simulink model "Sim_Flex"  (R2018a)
settings: Solver=ode113  StartTime=0.0  StopTime=20  FixedStep=0.0001  RelTol=1e-5  EnableMultiTasking=on
InitFcn:
  | init
StopFcn:
  | pl
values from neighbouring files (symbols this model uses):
  d2r = pi/180    (= 0.0174532925199)    [init.m]    (also in LQR_Design.m)
  Kr = Kq; Kr(3:4)=-Kq(3:4)    [init.m]
  Wf = 20    [init.m]
undefined symbols (not defined in the file or in its folder): Av, Bv, Cv, Dv, Kq, TVC
libraries: Actuator_Lib x16

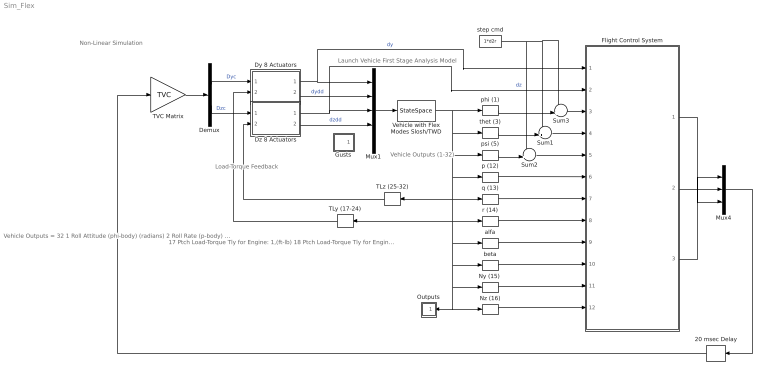
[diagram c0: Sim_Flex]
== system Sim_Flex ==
  note: Load-Torque Feedback
  note: 17 Ptch Load-Torque Tly for Engine: 1,(ft-lb) 18 Ptch Load-Torque Tly for Engine: 2,(ft-lb) 19 Ptch Load-Torque Tly for Engine: 3,(ft-lb) 20 Ptch Load-Torque Tly for Engine: 4,(ft-lb) 21 Ptch Load-Torque Tly for Engine: 5,(ft-lb) 22 Ptch Load-Torque Tly for Engine: 6,(ft-lb) 23 Ptch Load-Torque Tly for Engine: 7,(ft-lb) 24 Ptch Load-Torque Tly for Engine: 8,(ft-lb) 25 Yaw Load-Torque Tlz for Engine: 1,(ft-lb) 26 Yaw Load-Torque Tlz for Engine: 2,(ft-lb) 27 Yaw Load-Torque Tlz for Engine: 3,(ft-lb) 28 Yaw Load-Torque Tlz for Engine: 4,(ft-lb) 29 Yaw Load-Torque Tlz for Engine: 5,(ft-lb) 30 Yaw Load-Torque Tlz for Engine: 6,(ft-lb) 31 Yaw Load-Torque Tlz for Engine: 7,(ft-lb) 32 Yaw Load-Torque Tlz for Engine: 8,(ft-lb)
  note: Vehicle Outputs = 32 1 Roll Attitude (phi-body) (radians) 2 Roll Rate (p-body) (rad/sec) 3 Pitch Attitude (thet-bdy) (radians) 4 Pitch Rate (q-body) (rad/sec) 5 Yaw Attitude (psi-body) (radians) 6 Yaw Rate (r-body) (rad/sec) 7 Angle of attack, alfa, (radians) 8 Angle of sideslip, beta, (radian) 9 Change in Altitude, delta-h, (feet) 10 Forward Acceleration (V-dot) (ft/sec) 11 Cross Range Velocity (Vcr) (ft/sec) 12 Rate-Gyro # 1, Roll Rate (Body) (rad/sec) 13 Rate-Gyro # 2, Pitch Rate (Body) (rad/sec) 14 Rate-Gyro # 3, Yaw Rate (Body) (rad/sec) 15 Accelerom # 1, (along Y), (ft/sec^2) Translat. Accelerat. 16 Accelerom # 2, (along Z), (ft/sec^2) Translat. Accelerat.
  note: Vehicle Outputs (1-32)
  note: Non-Linear Simulation
  note: Launch Vehicle First Stage Analysis Model
  20 msec Delay : TransportDelay  DelayTime="[1  1  1]*0.02"  InitialOutput="[0  0  0]"  PadeOrder=2
  Demux : Demux  Outputs=[8, 8]
  Dy 8 Actuators : Subsystem
  Dz 8 Actuators : Subsystem
  Flight Control System : Subsystem
  Gusts : Subsystem
  Mux1 : Mux  Inputs=[8, 8, 8, 8, 1]
  Mux4 : Mux  Inputs=3
  "Ny (15) " : Selector  InputPortWidth=32  IndexOptions=Index vector (dialog)  Indices=[15]  OutputSizes=1
  Nz (16) : Selector  InputPortWidth=32  IndexOptions=Index vector (dialog)  Indices=[16]  OutputSizes=1
  Outputs : Subsystem
  Sum1 : Sum  Inputs=-+|
  Sum2 : Sum  Inputs=-+|
  Sum3 : Sum  Inputs=-+|
  TLy (17-24) : Selector  InputPortWidth=32  IndexOptions=Index vector (dialog)  Indices=[17:24]  OutputSizes=1
  TLz (25-32) : Selector  InputPortWidth=32  IndexOptions=Index vector (dialog)  Indices=[25:32]  OutputSizes=1
  TVC Matrix : Gain  Gain=TVC  Multiplication=Matrix(K*u)
  Vehicle with Flex Modes Slosh/TWD : StateSpace  A=Av  B=Bv  C=Cv  D=Dv  InitialCondition=0
  alfa : Selector  InputPortWidth=32  IndexOptions=Index vector (dialog)  Indices=[7]  OutputSizes=1
  beta : Selector  InputPortWidth=32  IndexOptions=Index vector (dialog)  Indices=[8]  OutputSizes=1
  p (12) : Selector  InputPortWidth=32  IndexOptions=Index vector (dialog)  Indices=[12]  OutputSizes=1
  phi (1) : Selector  InputPortWidth=32  IndexOptions=Index vector (dialog)  Indices=[1]  OutputSizes=1
  psi (5) : Selector  InputPortWidth=32  IndexOptions=Index vector (dialog)  Indices=[5]  OutputSizes=1
  q (13) : Selector  InputPortWidth=32  IndexOptions=Index vector (dialog)  Indices=[13]  OutputSizes=1
  r (14) : Selector  InputPortWidth=32  IndexOptions=Index vector (dialog)  Indices=[14]  OutputSizes=1
  step cmd : Constant  Value=1*d2r
  thet (3) : Selector  InputPortWidth=32  IndexOptions=Index vector (dialog)  Indices=[3]  OutputSizes=1
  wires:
  Mux1/1 -> Vehicle with Flex Modes Slosh/TWD/1
  Dy 8 Actuators/2(dydd) -> Mux1/2  "dydd"
  Dz 8 Actuators/2(dzdd) -> Mux1/4  "dzdd"
  Demux/1 -> Dy 8 Actuators/1(dy-com)  "Dyc"
  Dy 8 Actuators/1(DY) -> Flight Control System/1(dy), Mux1/1  "dy"
  Dz 8 Actuators/1(DZ) -> Flight Control System/2(dz), Mux1/3  "dz"
  Demux/2 -> Dz 8 Actuators/1(dz-com)  "Dzc"
  TLy (17-24)/1 -> Dy 8 Actuators/2(TLY)
  TLz (25-32)/1 -> Dz 8 Actuators/2(TLZ)
  Vehicle with Flex Modes Slosh/TWD/1 -> TLz (25-32)/1, "Ny (15) "/1, Outputs/1(in), Nz (16)/1, beta/1, alfa/1, TLy (17-24)/1, r (14)/1, q (13)/1, p (12)/1, psi (5)/1, thet (3)/1, phi (1)/1
  r (14)/1 -> Flight Control System/8(r)
  q (13)/1 -> Flight Control System/7(q)
  p (12)/1 -> Flight Control System/6(p)
  TVC Matrix/1 -> Demux/1
  alfa/1 -> Flight Control System/9(alfa)
  beta/1 -> Flight Control System/10(beta)
  "Ny (15) "/1 -> Flight Control System/11(NY)
  Nz (16)/1 -> Flight Control System/12(NZ)
  Flight Control System/2(DQ_tvc) -> Mux4/2
  Flight Control System/1(DP_tvc) -> Mux4/1
  Flight Control System/3(DR_tvc) -> Mux4/3
  Mux4/1 -> 20 msec Delay/1
  Sum3/1 -> Flight Control System/3(phi)
  phi (1)/1 -> Sum3/2
  Sum1/1 -> Flight Control System/4(thet)
  thet (3)/1 -> Sum1/2
  psi (5)/1 -> Sum2/2
  Sum2/1 -> Flight Control System/5(psi)
  step cmd/1 -> Sum3/1, Sum1/1, Sum2/1
  20 msec Delay/1 -> TVC Matrix/1

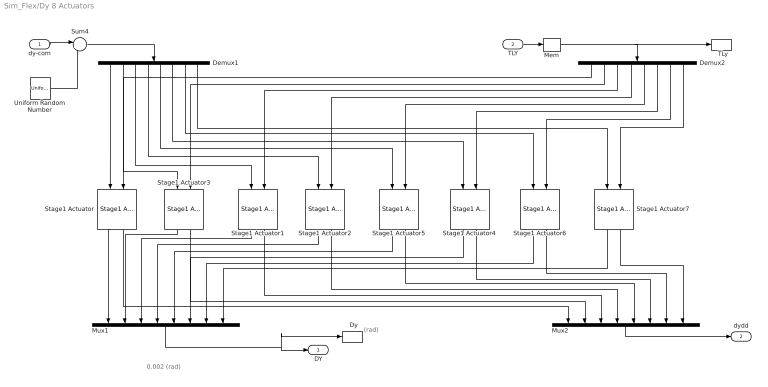
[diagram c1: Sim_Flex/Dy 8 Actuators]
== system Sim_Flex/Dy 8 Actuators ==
  note: (rad)
  note: 0.002 (rad)
  dy-com : Inport
  TLY : Inport  Port=2
  "  Dy" : ToWorkspace  VariableName=DY  SampleTime=-1
  "  TLy" : ToWorkspace  VariableName=TLy  SampleTime=-1
  Demux1 : Demux  Outputs=8
  Demux2 : Demux  Outputs=8
  Mem : Memory
  Mux1 : Mux  Inputs=8
  Mux2 : Mux  Inputs=8
  Stage1 Actuator{,1..7} (8 alike) : Actuator_Lib/Stage1 Actuator
  Sum4 : Sum  Inputs=|++
  Uniform Random Number : UniformRandomNumber  Minimum=[-1 -1 -1 -1 -1 -1 -1 -1]*0.002  Maximum=[1 1 1 1 1 1 1 1]*0.002  Seed=[10,11,12,13, 15,16,17,18]  SampleTime=0.001
  DY : Outport
  dydd : Outport  Port=2
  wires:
  Mux1/1 -> "  Dy"/1, DY/1
  TLY/1 -> Mem/1
  Mux2/1 -> dydd/1
  Stage1 Actuator2/1 -> Mux1/4
  Demux1/5 -> Stage1 Actuator5/1
  Stage1 Actuator4/2 -> Mux2/6
  Stage1 Actuator/1 -> Mux1/1
  Demux1/4 -> Stage1 Actuator2/1
  Stage1 Actuator7/1 -> Mux1/8
  Stage1 Actuator5/2 -> Mux2/5
  Stage1 Actuator5/1 -> Mux1/5
  Demux2/4 -> Stage1 Actuator2/2
  Demux2/6 -> Stage1 Actuator4/2
  Demux2/7 -> Stage1 Actuator6/2
  Stage1 Actuator1/2 -> Mux2/3
  Demux2/2 -> Stage1 Actuator3/2
  Stage1 Actuator2/2 -> Mux2/4
  Demux1/3 -> Stage1 Actuator1/1
  Stage1 Actuator6/2 -> Mux2/7
  Stage1 Actuator/2 -> Mux2/1
  Stage1 Actuator7/2 -> Mux2/8
  Stage1 Actuator3/2 -> Mux2/2
  Demux1/2 -> Stage1 Actuator3/1
  Demux1/7 -> Stage1 Actuator6/1
  Demux1/8 -> Stage1 Actuator7/1
  Stage1 Actuator3/1 -> Mux1/2
  Demux2/5 -> Stage1 Actuator5/2
  Demux1/1 -> Stage1 Actuator/1
  Demux2/1 -> Stage1 Actuator/2
  Stage1 Actuator6/1 -> Mux1/7
  Demux2/8 -> Stage1 Actuator7/2
  Demux2/3 -> Stage1 Actuator1/2
  Stage1 Actuator4/1 -> Mux1/6
  Stage1 Actuator1/1 -> Mux1/3
  Demux1/6 -> Stage1 Actuator4/1
  Mem/1 -> Demux2/1, "  TLy"/1
  dy-com/1 -> Sum4/1
  Uniform Random Number/1 -> Sum4/2
  Sum4/1 -> Demux1/1

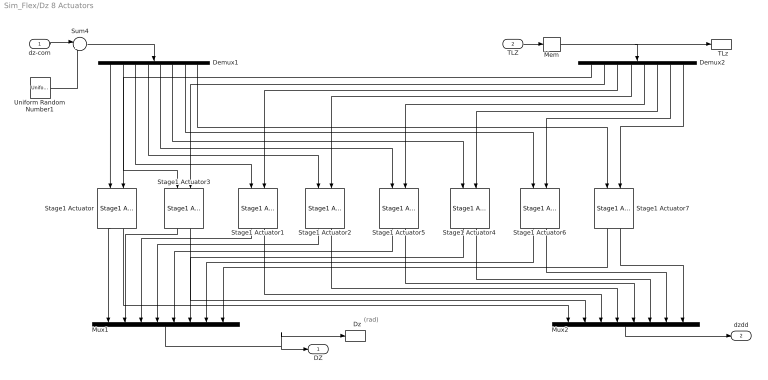
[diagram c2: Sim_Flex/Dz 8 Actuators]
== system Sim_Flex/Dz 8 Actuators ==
  note: (rad)
  dz-com : Inport
  TLZ : Inport  Port=2
  "  Dz" : ToWorkspace  VariableName=DZ  SampleTime=-1
  "  TLz" : ToWorkspace  VariableName=TLz  SampleTime=-1
  Demux1 : Demux  Outputs=8
  Demux2 : Demux  Outputs=8
  Mem : Memory
  Mux1 : Mux  Inputs=8
  Mux2 : Mux  Inputs=8
  Stage1 Actuator{,1..7} (8 alike) : Actuator_Lib/Stage1 Actuator
  Sum4 : Sum  Inputs=|++
  Uniform Random Number1 : UniformRandomNumber  Minimum=[-1 -1 -1 -1 -1 -1 -1 -1]*0.002  Maximum=[1 1 1 1 1 1 1 1]*0.002  Seed=[10,11,12,13, 15,16,17,18]  SampleTime=0.001
  DZ : Outport
  dzdd : Outport  Port=2
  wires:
  Mux1/1 -> "  Dz"/1, DZ/1
  TLZ/1 -> Mem/1
  Mux2/1 -> dzdd/1
  Stage1 Actuator2/1 -> Mux1/4
  Demux1/5 -> Stage1 Actuator5/1
  Stage1 Actuator4/2 -> Mux2/6
  Stage1 Actuator/1 -> Mux1/1
  Demux1/4 -> Stage1 Actuator2/1
  Stage1 Actuator7/1 -> Mux1/8
  Stage1 Actuator5/2 -> Mux2/5
  Stage1 Actuator5/1 -> Mux1/5
  Demux2/4 -> Stage1 Actuator2/2
  Demux2/6 -> Stage1 Actuator4/2
  Demux2/7 -> Stage1 Actuator6/2
  Stage1 Actuator1/2 -> Mux2/3
  Demux2/2 -> Stage1 Actuator3/2
  Stage1 Actuator2/2 -> Mux2/4
  Demux1/3 -> Stage1 Actuator1/1
  Stage1 Actuator6/2 -> Mux2/7
  Stage1 Actuator/2 -> Mux2/1
  Stage1 Actuator7/2 -> Mux2/8
  Stage1 Actuator3/2 -> Mux2/2
  Demux1/2 -> Stage1 Actuator3/1
  Demux1/7 -> Stage1 Actuator6/1
  Demux1/8 -> Stage1 Actuator7/1
  Stage1 Actuator3/1 -> Mux1/2
  Demux2/5 -> Stage1 Actuator5/2
  Demux1/1 -> Stage1 Actuator/1
  Demux2/1 -> Stage1 Actuator/2
  Stage1 Actuator6/1 -> Mux1/7
  Demux2/8 -> Stage1 Actuator7/2
  Demux2/3 -> Stage1 Actuator1/2
  Stage1 Actuator4/1 -> Mux1/6
  Stage1 Actuator1/1 -> Mux1/3
  Demux1/6 -> Stage1 Actuator4/1
  Mem/1 -> Demux2/1, "  TLz"/1
  dz-com/1 -> Sum4/1
  Uniform Random Number1/1 -> Sum4/2
  Sum4/1 -> Demux1/1

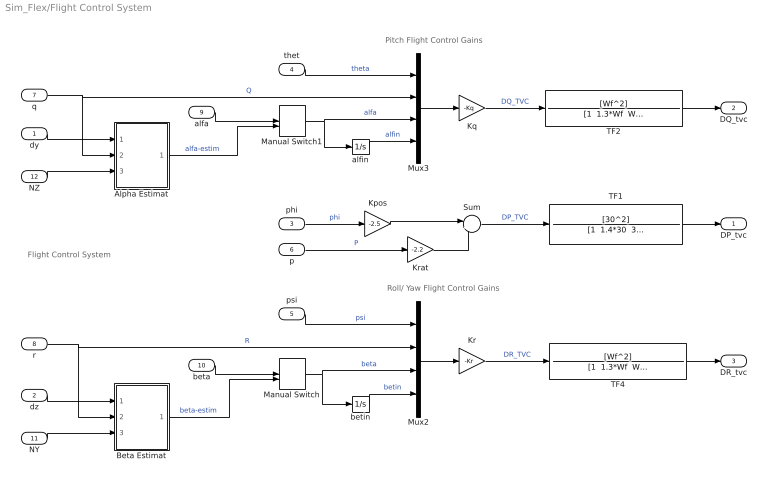
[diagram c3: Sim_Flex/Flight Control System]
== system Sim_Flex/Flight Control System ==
  note: Pitch Flight Control Gains
  note: Roll/ Yaw Flight Control Gains
  note: Flight Control System
  dy : Inport
  dz : Inport  Port=2
  phi : Inport  Port=3
  thet : Inport  Port=4
  psi : Inport  Port=5
  p : Inport  Port=6
  q : Inport  Port=7
  r : Inport  Port=8
  alfa : Inport  Port=9
  beta : Inport  Port=10
  NY : Inport  Port=11
  NZ : Inport  Port=12
  Alpha Estimat : Subsystem
  Beta Estimat : Subsystem
  Kpos : Gain  Gain=-2.5  Multiplication=Matrix(K*u)
  Kq : Gain  Gain=-Kq  Multiplication=Matrix(K*u)
  Kr : Gain  Gain=-Kr  Multiplication=Matrix(K*u)
  Krat : Gain  Gain=-2.2  Multiplication=Matrix(K*u)
  Manual Switch : ManualSwitch  CurrentSetting=0
  Manual Switch1 : ManualSwitch  CurrentSetting=0
  Mux2 : Mux
  Mux3 : Mux
  Sum : Sum  Inputs=|++
  TF1 : TransferFcn  Numerator=[30^2]  Denominator="[1  1.4*30  30^2]"
  TF2 : TransferFcn  Numerator=[Wf^2]  Denominator="[1  1.3*Wf  Wf^2]"
  TF4 : TransferFcn  Numerator=[Wf^2]  Denominator="[1  1.3*Wf  Wf^2]"
  alfin : Integrator
  betin : Integrator
  DP_tvc : Outport
  DQ_tvc : Outport  Port=2
  DR_tvc : Outport  Port=3
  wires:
  Alpha Estimat/1(alfest) -> Manual Switch1/2  "alfa-estim"
  alfa/1 -> Manual Switch1/1
  Manual Switch1/1 -> Mux3/3, alfin/1  "alfa"
  beta/1 -> Manual Switch/1
  Manual Switch/1 -> betin/1, Mux2/3  "beta"
  psi/1 -> Mux2/1  "psi"
  betin/1 -> Mux2/4  "betin"
  q/1 -> Alpha Estimat/2(q), Mux3/2  "Q"
  r/1 -> Mux2/2, Beta Estimat/2(r)  "R"
  alfin/1 -> Mux3/4  "alfin"
  thet/1 -> Mux3/1  "theta"
  Kq/1 -> TF2/1  "DQ_TVC"
  NZ/1 -> Alpha Estimat/3(Zdd)
  NY/1 -> Beta Estimat/3(Ydd)
  Beta Estimat/1(betest) -> Manual Switch/2  "beta-estim"
  dy/1 -> Alpha Estimat/1(dy)
  dz/1 -> Beta Estimat/1(dz)
  Mux3/1 -> Kq/1
  Kpos/1 -> Sum/1
  Sum/1 -> TF1/1  "DP_TVC"
  Krat/1 -> Sum/2
  p/1 -> Krat/1  "P"
  phi/1 -> Kpos/1  "phi"
  Mux2/1 -> Kr/1
  TF1/1 -> DP_tvc/1
  TF2/1 -> DQ_tvc/1
  Kr/1 -> TF4/1  "DR_TVC"
  TF4/1 -> DR_tvc/1

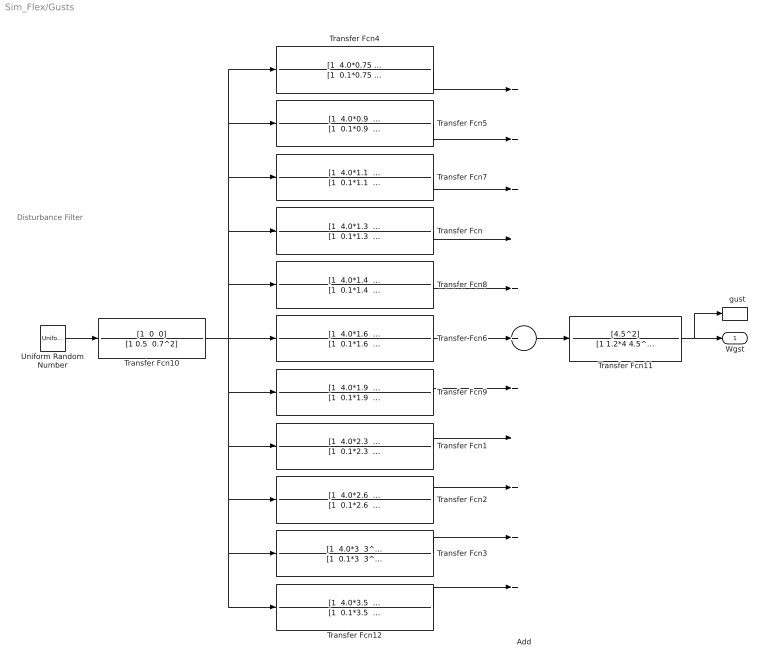
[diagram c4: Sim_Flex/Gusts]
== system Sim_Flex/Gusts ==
  note: Disturbance Filter
  "  gust" : ToWorkspace  VariableName=Wgst  SampleTime=-1
  Add : Sum  Inputs=+++++++++++
  Transfer Fcn : TransferFcn  Numerator="[1  4.0*1.3  1.3^2]"  Denominator="[1  0.1*1.3  1.3^2]"
  Transfer Fcn1 : TransferFcn  Numerator="[1  4.0*2.3  2.3^2]"  Denominator="[1  0.1*2.3  2.3^2]"
  Transfer Fcn10 : TransferFcn  Numerator="[1  0  0]"  Denominator="[1 0.5  0.7^2]"
  Transfer Fcn11 : TransferFcn  Numerator=[4.5^2]  Denominator=[1 1.2*4 4.5^2]
  Transfer Fcn12 : TransferFcn  Numerator="[1  4.0*3.5  3.5^2]"  Denominator="[1  0.1*3.5  3.5^2]"
  Transfer Fcn2 : TransferFcn  Numerator="[1  4.0*2.6  2.6^2]"  Denominator="[1  0.1*2.6  2.6^2]"
  Transfer Fcn3 : TransferFcn  Numerator="[1  4.0*3  3^2]"  Denominator="[1  0.1*3  3^2]"
  Transfer Fcn4 : TransferFcn  Numerator="[1  4.0*0.75  0.75^2]"  Denominator="[1  0.1*0.75  0.75^2]"
  Transfer Fcn5 : TransferFcn  Numerator="[1  4.0*0.9  0.9^2]"  Denominator="[1  0.1*0.9  0.9^2]"
  Transfer Fcn6 : TransferFcn  Numerator="[1  4.0*1.6  1.6^2]"  Denominator="[1  0.1*1.6  1.6^2]"
  Transfer Fcn7 : TransferFcn  Numerator="[1  4.0*1.1  1.1^2]"  Denominator="[1  0.1*1.1  1.1^2]"
  Transfer Fcn8 : TransferFcn  Numerator="[1  4.0*1.4  1.4^2]"  Denominator="[1  0.1*1.4  1.4^2]"
  Transfer Fcn9 : TransferFcn  Numerator="[1  4.0*1.9  1.9^2]"  Denominator="[1  0.1*1.9  1.9^2]"
  Uniform Random Number : UniformRandomNumber  SampleTime=0.1
  Wgst : Outport
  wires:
  Transfer Fcn9/1 -> Add/7
  Transfer Fcn8/1 -> Add/5
  Transfer Fcn2/1 -> Add/9
  Transfer Fcn10/1 -> Transfer Fcn9/1, Transfer Fcn3/1, Transfer Fcn12/1, Transfer Fcn2/1, Transfer Fcn1/1, Transfer Fcn8/1, Transfer Fcn/1, Transfer Fcn7/1, Transfer Fcn4/1, Transfer Fcn5/1, Transfer Fcn6/1
  Transfer Fcn1/1 -> Add/8
  Transfer Fcn7/1 -> Add/3
  Add/1 -> Transfer Fcn11/1
  Transfer Fcn/1 -> Add/4
  Transfer Fcn4/1 -> Add/1
  Transfer Fcn5/1 -> Add/2
  Transfer Fcn6/1 -> Add/6
  Transfer Fcn11/1 -> Wgst/1, "  gust"/1
  Transfer Fcn3/1 -> Add/10
  Transfer Fcn12/1 -> Add/11
  Uniform Random Number/1 -> Transfer Fcn10/1

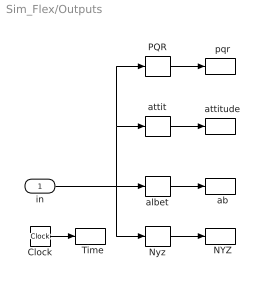
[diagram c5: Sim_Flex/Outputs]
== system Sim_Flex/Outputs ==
  in : Inport
  "  NYZ" : ToWorkspace  VariableName=Nyz  SampleTime=-1
  "  Time" : ToWorkspace  VariableName=tim  SampleTime=-1
  "  ab" : ToWorkspace  VariableName=albet  SampleTime=-1
  "  attitude" : ToWorkspace  VariableName=atti  SampleTime=-1
  "  pqr" : ToWorkspace  VariableName=pqr  SampleTime=-1
  Clock : Clock
  Nyz : Selector  InputPortWidth=32  IndexOptions=Index vector (dialog)  Indices=[15,16]  OutputSizes=1
  PQR : Selector  InputPortWidth=32  IndexOptions=Index vector (dialog)  Indices=[12, 13, 14]  OutputSizes=1
  albet : Selector  InputPortWidth=32  IndexOptions=Index vector (dialog)  Indices=[7,8]  OutputSizes=1
  attit : Selector  InputPortWidth=32  IndexOptions=Index vector (dialog)  Indices="[1  3   5]"  OutputSizes=1
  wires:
  PQR/1 -> "  pqr"/1
  Clock/1 -> "  Time"/1
  albet/1 -> "  ab"/1
  attit/1 -> "  attitude"/1
  in/1 -> albet/1, Nyz/1, attit/1, PQR/1
  Nyz/1 -> "  NYZ"/1

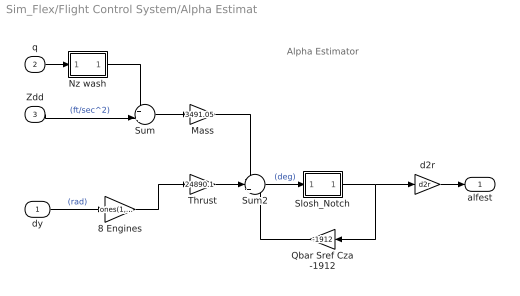
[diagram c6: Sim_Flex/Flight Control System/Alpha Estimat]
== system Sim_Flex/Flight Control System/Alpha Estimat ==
  note: Alpha Estimator
  dy : Inport
  q : Inport  Port=2
  Zdd : Inport  Port=3
  8 Engines : Gain  Gain=ones(1,8)  Multiplication=Matrix(K*u) (u vector)
  Mass : Gain  Gain=3491.05
  Nz wash : Subsystem
  Qbar Sref Cza -1912 : Gain  Gain=-1912
  Slosh_Notch : Subsystem
  Sum : Sum  Inputs=++|
  Sum2 : Sum  Inputs=--+
  Thrust : Gain  Gain=24890.1
  d2r : Gain  Gain=d2r
  alfest : Outport
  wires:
  dy/1 -> 8 Engines/1  "(rad)"
  Sum/1 -> Mass/1
  q/1 -> Nz wash/1(in)
  d2r/1 -> alfest/1
  Zdd/1 -> Sum/2  "(ft/sec^2)"
  Qbar Sref Cza -1912/1 -> Sum2/3
  Sum2/1 -> Slosh_Notch/1(in)  "(deg)"
  Nz wash/1(ou) -> Sum/1
  Slosh_Notch/1(ou) -> d2r/1, Qbar Sref Cza -1912/1
  Mass/1 -> Sum2/1
  Thrust/1 -> Sum2/2
  8 Engines/1 -> Thrust/1

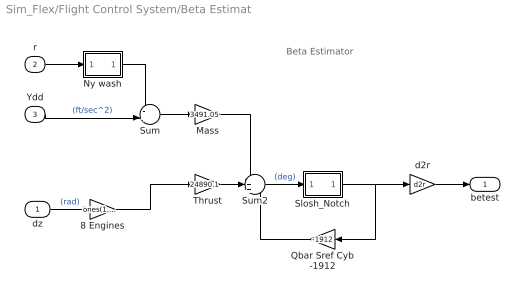
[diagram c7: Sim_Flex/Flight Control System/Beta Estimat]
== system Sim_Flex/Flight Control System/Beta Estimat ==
  note: Beta Estimator
  dz : Inport
  r : Inport  Port=2
  Ydd : Inport  Port=3
  8 Engines : Gain  Gain=ones(1,8)  Multiplication=Matrix(K*u) (u vector)
  Mass : Gain  Gain=3491.05
  Ny wash : Subsystem
  Qbar Sref Cyb -1912 : Gain  Gain=-1912
  Slosh_Notch : Subsystem
  Sum : Sum  Inputs=-+|
  Sum2 : Sum  Inputs=-++
  Thrust : Gain  Gain=24890.1
  d2r : Gain  Gain=d2r
  betest : Outport
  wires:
  Sum/1 -> Mass/1
  r/1 -> Ny wash/1(in)
  Thrust/1 -> Sum2/2
  d2r/1 -> betest/1
  Mass/1 -> Sum2/1
  Ydd/1 -> Sum/2  "(ft/sec^2)"
  Qbar Sref Cyb -1912/1 -> Sum2/3
  Sum2/1 -> Slosh_Notch/1(in)  "(deg)"
  Ny wash/1(ou) -> Sum/1
  Slosh_Notch/1(ou) -> Qbar Sref Cyb -1912/1, d2r/1
  dz/1 -> 8 Engines/1  "(rad)"
  8 Engines/1 -> Thrust/1

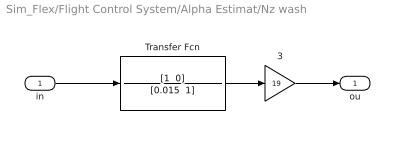
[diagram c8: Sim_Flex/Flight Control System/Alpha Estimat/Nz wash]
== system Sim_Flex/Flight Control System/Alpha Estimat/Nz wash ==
  in : Inport
  3 : Gain  Gain=19
  Transfer Fcn : TransferFcn  Numerator="[1  0]"  Denominator="[0.015  1]"
  ou : Outport
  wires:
  in/1 -> Transfer Fcn/1
  Transfer Fcn/1 -> 3/1
  3/1 -> ou/1

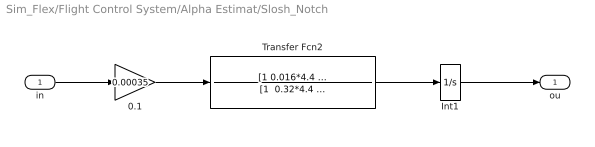
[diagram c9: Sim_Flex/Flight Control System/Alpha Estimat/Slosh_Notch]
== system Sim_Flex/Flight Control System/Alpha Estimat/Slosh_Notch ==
  in : Inport
  0.1 : Gain  Gain=0.00035
  Int1 : Integrator
  Transfer Fcn2 : TransferFcn  Numerator="[1 0.016*4.4  4.38^2]"  Denominator="[1  0.32*4.4  4.38^2]"
  ou : Outport
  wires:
  in/1 -> 0.1/1
  Transfer Fcn2/1 -> Int1/1
  0.1/1 -> Transfer Fcn2/1
  Int1/1 -> ou/1

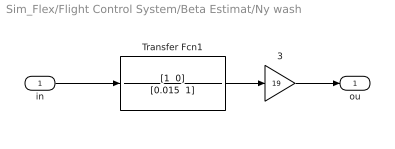
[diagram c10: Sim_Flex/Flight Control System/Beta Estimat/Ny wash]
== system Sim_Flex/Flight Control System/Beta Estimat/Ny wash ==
  in : Inport
  3 : Gain  Gain=19
  Transfer Fcn1 : TransferFcn  Numerator="[1  0]"  Denominator="[0.015  1]"
  ou : Outport
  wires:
  in/1 -> Transfer Fcn1/1
  Transfer Fcn1/1 -> 3/1
  3/1 -> ou/1

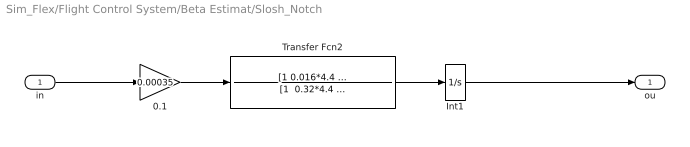
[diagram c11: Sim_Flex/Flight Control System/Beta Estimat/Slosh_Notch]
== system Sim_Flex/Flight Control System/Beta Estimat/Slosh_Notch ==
  in : Inport
  0.1 : Gain  Gain=0.00035
  Int1 : Integrator
  Transfer Fcn2 : TransferFcn  Numerator="[1 0.016*4.4  4.38^2]"  Denominator="[1  0.32*4.4  4.38^2]"
  ou : Outport
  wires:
  in/1 -> 0.1/1
  Int1/1 -> ou/1
  0.1/1 -> Transfer Fcn2/1
  Transfer Fcn2/1 -> Int1/1
